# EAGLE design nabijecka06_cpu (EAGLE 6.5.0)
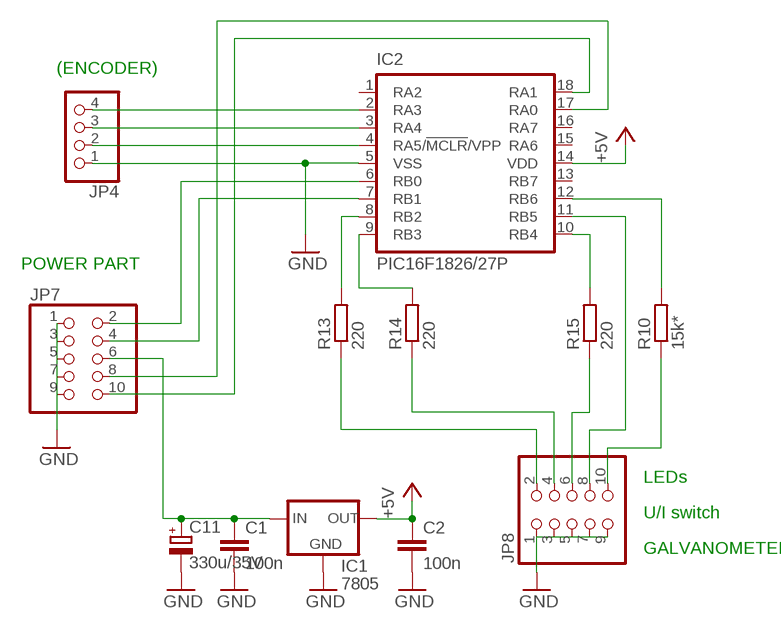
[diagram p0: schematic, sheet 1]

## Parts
C1  100n  C-EU050-024X044  [C050-024X044]
C2  100n  C-EU050-024X044  [C050-024X044]
C11  330u/35V  CPOL-EUE5-8.5  [E5-8,5]
IC1  7805  78XXL  [78XXL]
IC2  PIC16F1826/27P  [DIL18]
JP4  PINHD-1X4  [1X04]
JP7  PINHD-2X5  [2X05]
JP8  PINHD-2X5  [2X05]
R10  15k*  R-EU_0204/7  [0204/7]
R13  220  R-EU_0204/7  [0204/7]
R14  220  R-EU_0204/7  [0204/7]
R15  220  R-EU_0204/7  [0204/7]

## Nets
+5V: C2.1 IC1.OUT IC2.14(VDD)
G+: JP8.10 R10.1
GND: C1.2 C2.2 C11.- IC1.GND IC2.5(VSS) JP4.1 JP7.1 JP7.3 JP7.5 JP7.7 JP7.9 JP8.1 JP8.3 JP8.5 JP8.7 JP8.9
N$1: JP8.2 R13.1
N$2: JP8.4 R14.1
N$3: JP8.6 R15.1
N$7: IC2.6(RB0) JP7.2
N$8: IC2.7(RB1) JP7.4
N$10: IC2.18(RA1) JP7.10
N$11: IC2.17(RA0) JP7.8
N$12: IC2.12(RB6) R10.2
N$13: IC2.4(RA5/!MCLR!/VPP) JP4.2
N$21: IC2.8(RB2) R13.2
N$25: IC2.9(RB3) R14.2
N$26: IC2.10(RB4) R15.2
N$29: IC2.3(RA4) JP4.3
N$30: IC2.2(RA3) JP4.4
N$33: IC2.11(RB5) JP8.8
VCC: C1.1 C11.+ IC1.IN JP7.6
Unconnected: IC2.1(RA2) IC2.13(RB7) IC2.15(RA6) IC2.16(RA7)

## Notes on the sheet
- (ENCODER)
- POWER PART
- LEDs
- U/I switch
- GALVANOMETER

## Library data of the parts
C1 C2 = rcl:C-EU: CAPACITOR, European symbol
C11 = rcl:CPOL-EU: POLARIZED CAPACITOR, European symbol
IC1 = v-reg:78XXL: VOLTAGE REGULATOR
IC2 = microchip:PIC16*F1826/27: 18/20/28-Pin Flash Microcontrollers with nanoWatt XLP Technology Source: www.microchip.com PIC16F1827.pdf
JP4 = pinhead:PINHD-1X4: PIN HEADER
JP7 JP8 = pinhead:PINHD-2X5: PIN HEADER
R10 R13-R15 = rcl:R-EU_: RESISTOR, European symbol

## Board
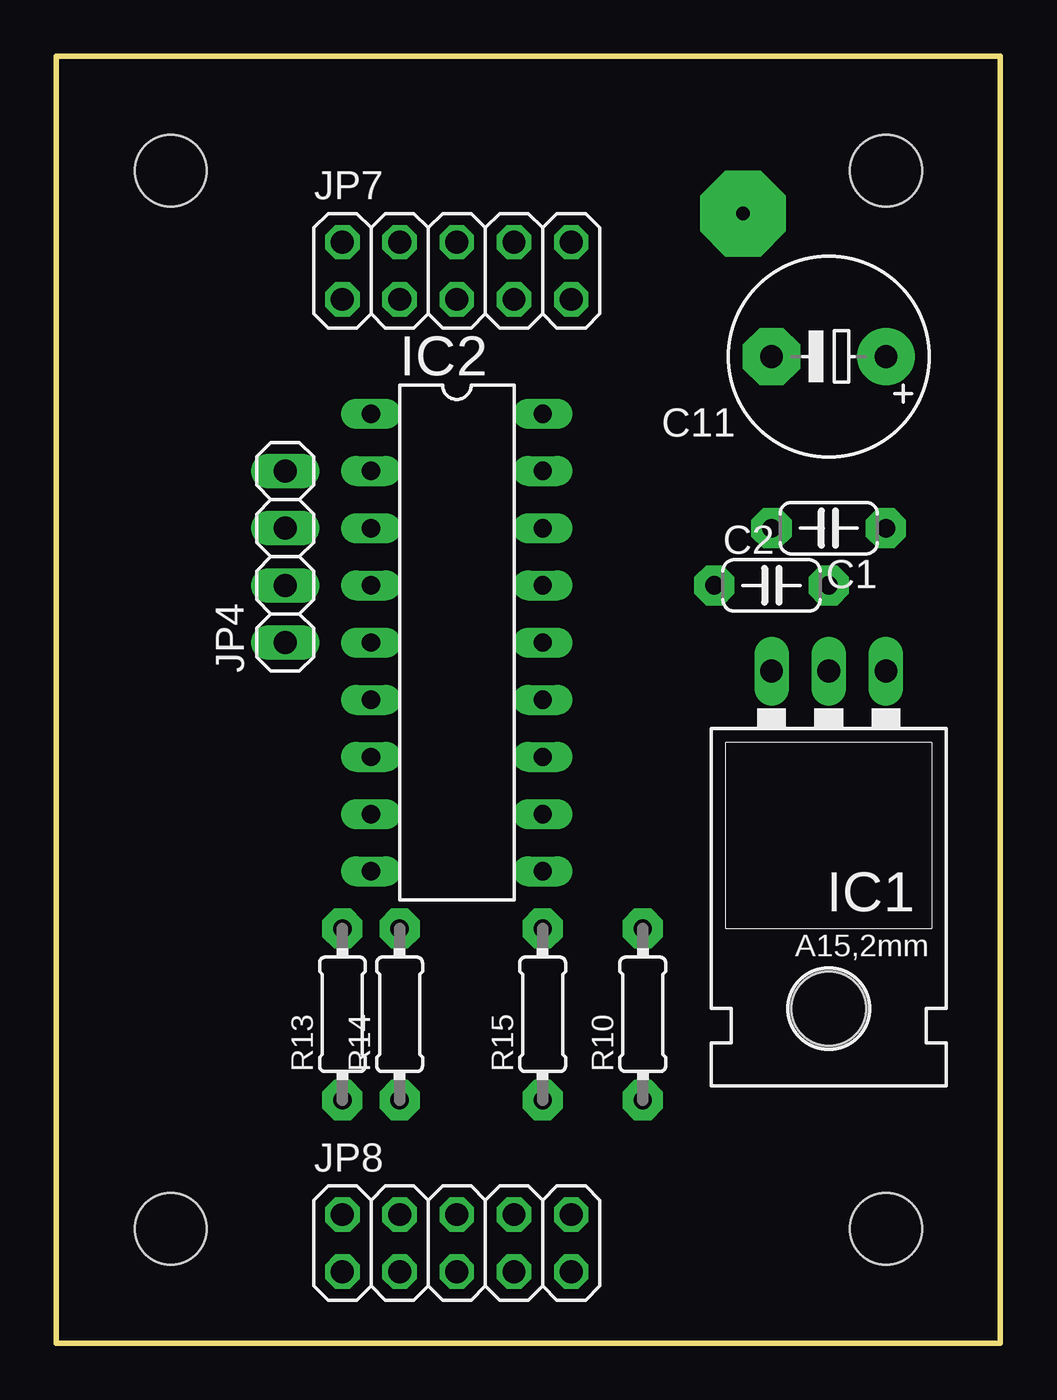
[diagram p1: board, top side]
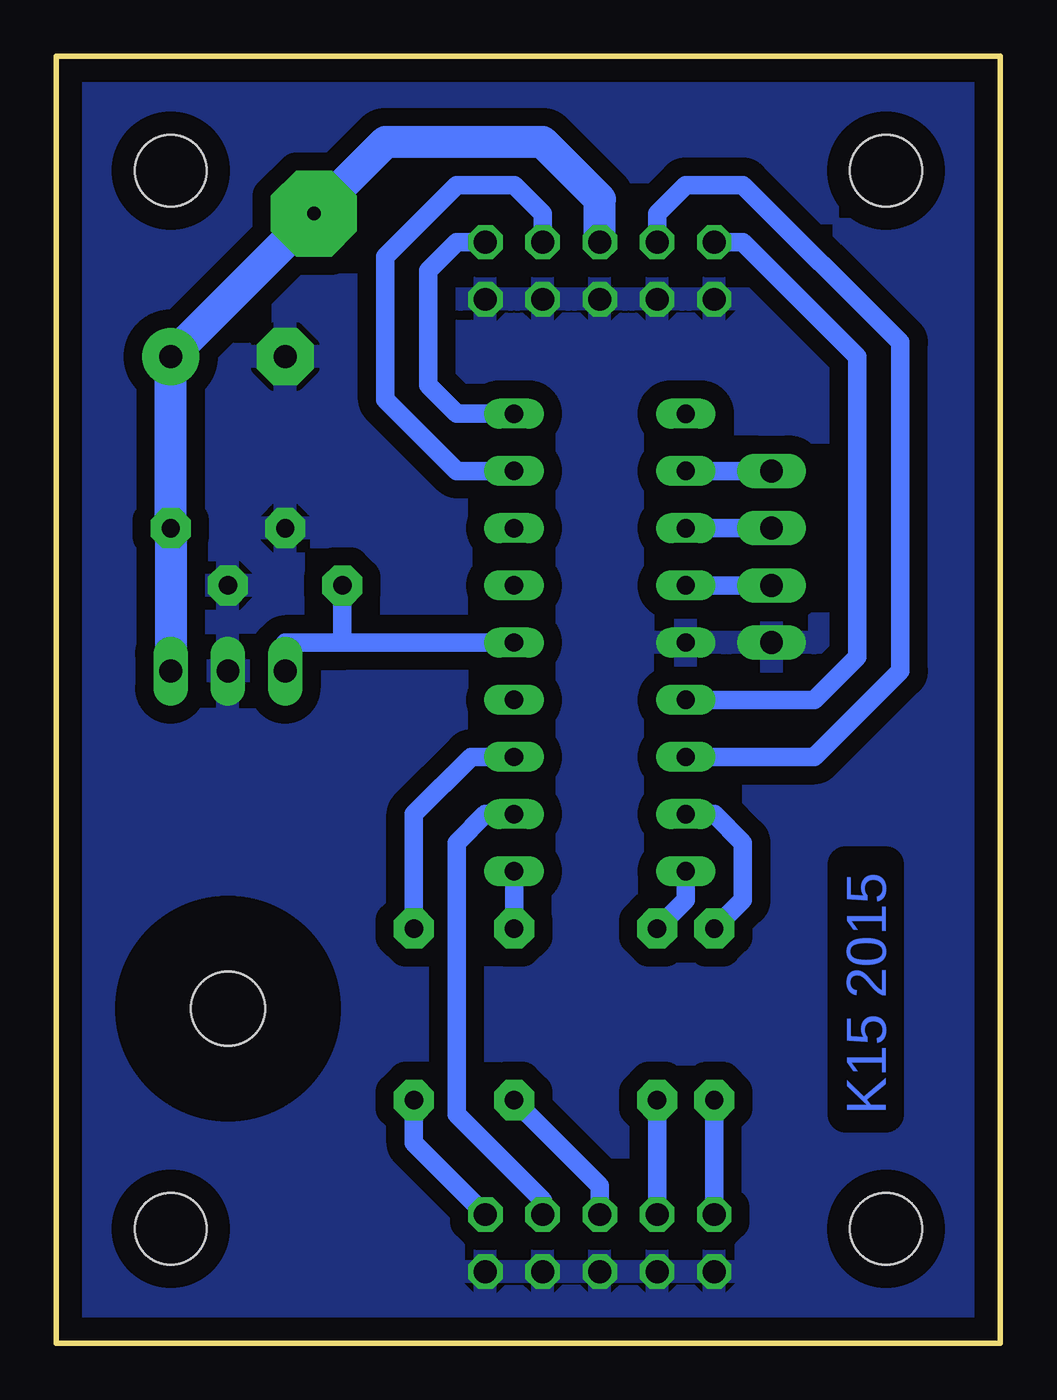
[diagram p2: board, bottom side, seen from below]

Size 41.91 x 57.15 mm. Coordinates in mm from the lower left corner, seen from the top.
Outline: 0,0 0,57.15 41.91,57.15 41.91,0 0,0
Copper layers (1*16): Top 0.035mm / dielectric 1.5mm / Bottom 0.035mm
Design rules "default": minimum track width 10mil, minimum drill 24mil, track to track 8mil, track to pad 8mil, pad to pad 8mil, via to via 8mil, smd to smd 8mil, copper to edge 40mil, drill to drill 8mil, minimum pad ring 10mil, minimum via ring 8mil, stop-mask expansion 4mil, vias tented up to drill 0mil, thermal gap 10mil
Holes 3.2 mm at 5.08,52.07 5.08,5.08 36.83,5.08 36.83,52.07

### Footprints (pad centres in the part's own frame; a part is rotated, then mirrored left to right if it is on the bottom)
C050-024X044 = drill 0.813 pad 1.778 octagon: 1 -2.54,0; 2 2.54,0
E5-8,5 = drill 1.016 pad 2.54: + -2.54,0 | drill 1.016 pad 2.54 octagon: - 2.54,0
78XXL = drill 1.016 long: GND 0,-3.81; IN -2.54,-3.81; OUT 2.54,-3.81 | hole 3.302: 0,11.176
DIL18 = drill 0.813 long: 1 -10.16,-3.81; 2 -7.62,-3.81; 3 -5.08,-3.81; 4 -2.54,-3.81; 5 0,-3.81; 6 2.54,-3.81; 7 5.08,-3.81; 8 7.62,-3.81; 9 10.16,-3.81; 10 10.16,3.81; 11 7.62,3.81; 12 5.08,3.81; 13 2.54,3.81; 14 0,3.81; 15 -2.54,3.81; 16 -5.08,3.81; 17 -7.62,3.81; 18 -10.16,3.81
1X04 = drill 1.016 long: 1 -3.81,0; 2 -1.27,0; 3 1.27,0; 4 3.81,0
2X05 = drill 1.016 octagon: 1 -5.08,-1.27; 2 -5.08,1.27; 3 -2.54,-1.27; 4 -2.54,1.27; 5 0,-1.27; 6 0,1.27; 7 2.54,-1.27; 8 2.54,1.27; 9 5.08,-1.27; 10 5.08,1.27
0204/7 = drill 0.813 pad 1.778 octagon: 1 -3.81,0; 2 3.81,0

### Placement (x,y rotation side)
C1  34.29,36.2 180 top
C2  31.75,33.66 0 top
C11  34.29,43.81 180 top
IC1  34.29,26.04 180 top
IC2  17.78,31.11 270 top
JP4  10.16,34.92 90 top
JP7  17.78,47.62 0 top
JP8  17.78,4.45 0 top
R10  26.04,14.61 90 top
R13  12.7,14.61 90 top
R14  15.24,14.61 90 top
R15  21.59,14.61 90 top

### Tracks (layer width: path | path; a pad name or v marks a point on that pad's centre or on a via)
+5V
  Bottom 0.813: IC2.14 29.21,31.11 | 29.21,31.11 31.75,31.11 IC1.OUT | C2.1 29.21,31.11
G+
  Bottom 0.813: JP8.10 26.04,8.89 R10.1
GND
  pour Bottom (isolate 0.813): 0,57.15 41.91,57.15 41.91,-1.27 0,-1.27
N$1
  Bottom 0.813: JP8.2 R13.1
N$2
  Bottom 0.813: JP8.4 R14.1
N$3
  Bottom 0.813: JP8.6 17.78,6.99 R15.1
N$7
  Bottom 0.813: IC2.6 8.26,28.57 6.35,30.48 6.35,43.81 11.43,48.89 JP7.2
N$8
  Bottom 0.813: IC2.7 8.26,26.04 4.45,29.84 4.45,44.45 11.43,51.44 13.97,51.44 15.24,50.16 JP7.4
N$10
  Bottom 0.813: IC2.18 24.13,41.27 25.4,42.55 25.4,47.62 24.13,48.89 JP7.10
N$11
  Bottom 0.813: IC2.17 24.13,38.73 27.3,41.91 27.3,48.26 24.13,51.44 21.59,51.44 20.32,50.16 JP7.8
N$12
  Bottom 0.813: R10.2 26.04,23.49 23.5,26.04 IC2.12
N$13
  Bottom 0.813: JP4.2 IC2.4
N$21
  Bottom 0.813: IC2.8 12.7,23.49 11.43,22.22 11.43,19.68 R13.2
N$25
  Bottom 0.813: IC2.9 13.97,19.68 R14.2
N$26
  Bottom 0.813: IC2.10 R15.2
N$29
  Bottom 0.813: JP4.3 IC2.3
N$30
  Bottom 0.813: JP4.4 IC2.2
N$33
  Bottom 0.813: IC2.11 22.86,23.49 24.13,22.22 24.13,10.16 20.32,6.35 JP8.8
VCC  (via drill 0.6 pad 3.81)
  Bottom 1.422: IC1.IN C1.1 C11.+ v30.48,50.16 27.3,53.34 20.32,53.34 17.78,50.8 JP7.6

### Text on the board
Bottom: K15 2015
